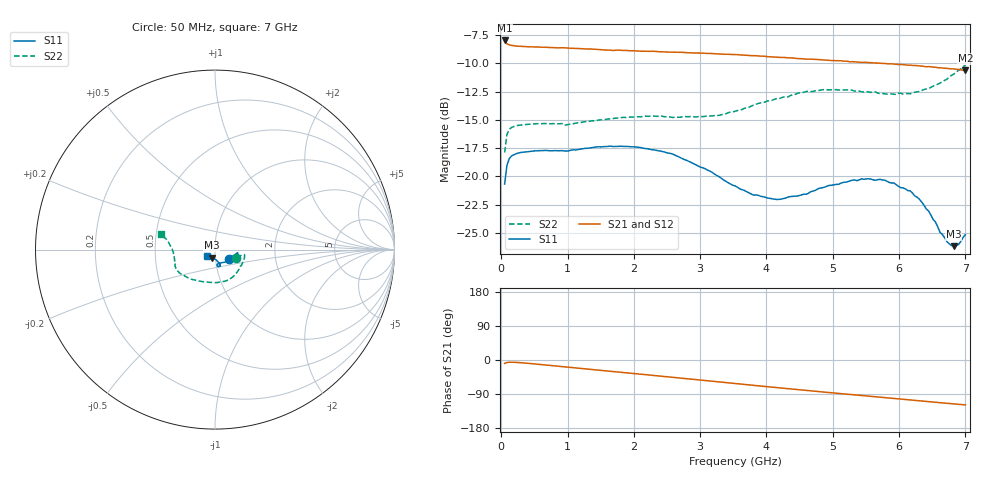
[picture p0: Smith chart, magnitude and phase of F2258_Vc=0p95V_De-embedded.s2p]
! Integrated Device Technology
! Corporate Headquarters
! 6024 Silver Creek Valley Road
! San Jose, CA 95138  USA
! Phone:  1-408-284-8200
! Toll Free:  1-800-223-1366
! Webpage:  http://www.idt.com/
! Timing and RF Division
! 515 Groton Road, Suite 102
! Westford, MA 01886-6024
! Device:  F2258
! Description: Voltage Variable RF Attenuator
! Frequency:  50.0 -  6000.00 MHz
! Package:  3x3 mm Thin QFN Plastic Package: 16 pin
! Ports:  2 RF, 2 DC
!  Pin  1  = NC
!  Pin  2  = NC
!  Pin  3  = RF2  = Port 2
!  Pin  4  = GND
!  Pin  5  = Vdd
!  Pin  6  = NC
!  Pin  7  = VCTRL
!  Pin  8  = NC
!  Pin  9  = GND
!  Pin 10  = RF1  = Port 1
!  Pin 11  = NC
!  Pin 12  = NC
!  Pin 13  = NC
!  Pin 14  = NC
!  Pin 15  = NC
!  Pin 16  = NC
! Vcntrl:  0.950 Volts
! Vdd:  +3.300 Volts
! Current:  1.150 mA
! Data:  The device was measured on a the F2258 evaluation board which has
!  individual transmission lines to the RF pins.  Data was collected
!  using a calibrated network analyzer.  The evaluation board was
!  de-embedded using a TRL calibration technique.
!  The reference plane is the edge of the package pin.
! Misc:  SN 10
!  Action Tracker AT0285
! Date Measured:  2014-12-10
! Date:  2016-01-13  MJV
! Note:
!  Integrated Device Technology supplies this data as a sample of measured
!  data at the package pin for this product.  Your particular data for this
!  product may vary.
!  Data was taken at 25 degrees C.
!  Integrated Device Technology reserves the right to change this data at anytime.
!Freq_(GHz)  S11M_(dB)  S11P_(deg)  S21M_(dB)  S21P_(deg)  S12M_(dB)  S12P_(deg)  S22M_(dB)  S22P_(deg)
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# GHz S dB R 50
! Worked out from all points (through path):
!   201 points, 50 MHz to 7 GHz, reference 50 ohm
!   highest |S21| = -7.98 dB at 50 MHz (marker M1); lowest = -10.6 dB at 7 GHz (marker M2)
!   group delay of S21, straight-line fit = 46.5 ps
!   lowest |S11| = -26.2 dB at 6.826 GHz (marker M3), VSWR 1.10, Z = 48 - j4.39 ohm
!   |S11| at or under -10 dB: start of sweep to end of sweep
!   |S22| runs from -17.9 to -10.1 dB; largest |S21 - S12| = 0.0016
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0.05  -20.68 -34.3  -7.98 -9.0  -7.98 -9.0  -17.89 -20.4
0.08475  -19.03 -16.4  -8.28 -6.6  -8.28 -6.6  -16.30 -11.3
0.1195  -18.43 -11.2  -8.37 -5.9  -8.38 -5.9  -15.84 -9.7
0.189  -18.08 -8.5  -8.45 -6.0  -8.46 -6.0  -15.59 -9.9
1.2315  -17.56 -20.5  -8.72 -22.8  -8.74 -22.8  -15.19 -41.6
1.82225  -17.33 -25.1  -8.86 -32.7  -8.86 -32.7  -14.79 -57.7
2.37825  -17.74 -28.4  -8.98 -42.1  -8.99 -42.1  -14.67 -73.1
3.07325  -19.31 -37.4  -9.11 -54.1  -9.12 -54.1  -14.69 -96.9
3.525  -20.84 -49.4  -9.23 -62.0  -9.24 -62.0  -14.24 -115.0
3.803  -21.64 -60.5  -9.32 -66.8  -9.33 -66.8  -13.70 -125.5
4.1505  -22.03 -71.8  -9.46 -72.7  -9.47 -72.7  -13.13 -135.9
4.7065  -21.29 -81.9  -9.64 -82.0  -9.65 -82.0  -12.47 -148.5
5.43625  -20.20 -77.1  -9.92 -93.7  -9.91 -93.7  -12.52 -160.3
5.85325  -20.54 -72.0  -10.05 -100.4  -10.04 -100.4  -12.70 -168.8
6.166  -21.27 -71.2  -10.16 -105.4  -10.18 -105.4  -12.69 -176.1
6.305  -22.00 -72.8  -10.23 -107.7  -10.24 -107.6  -12.49 -179.8
6.54825  -24.02 -80.3  -10.35 -111.5  -10.36 -111.5  -11.94 173.8
6.61775  -24.94 -84.7  -10.40 -112.5  -10.40 -112.6  -11.75 171.9
6.722  -25.77 -96.0  -10.45 -114.2  -10.46 -114.3  -11.41 169.2
6.82625  -26.16 -111.9  -10.50 -115.8  -10.50 -115.9  -10.95 167.3
6.89575  -26.02 -124.5  -10.55 -116.9  -10.55 -117.0  -10.61 165.8
7  -25.15 -141.1  -10.64 -118.4  -10.61 -118.5  -10.14 163.9
